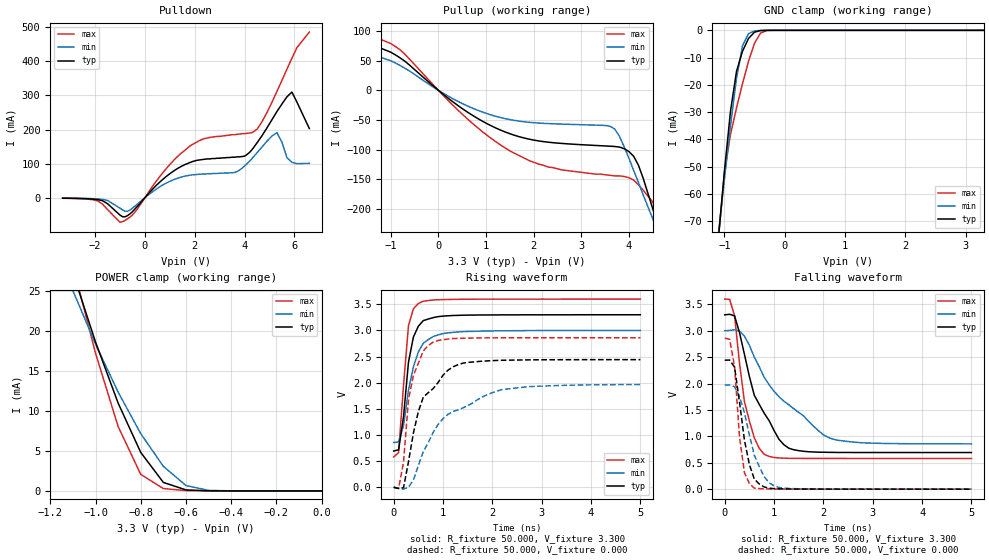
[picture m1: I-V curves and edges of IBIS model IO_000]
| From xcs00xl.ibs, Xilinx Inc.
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|   Model IO_000
[Model]   IO_000
Model_type   I/O
Polarity   Non-Inverting
Enable   Active-Low
Vinl =   0.800V
Vinh =   2.000V
Vmeas =   1.650V
Cref =  50.000pF
Rref =   1.000M
Vref =  0.000V
C_comp   5.300pF   3.500pF   6.800pF
[Temperature Range]   50.000   100.000   0.000
[Voltage Range]   3.300V   3.000V   3.600V
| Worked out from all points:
|   slope of the pulldown table from 0 to 0.495 V, typ, clamps not added: 12.8 ohm
|   slope of the pullup table from 0 to 0.495 V, typ, clamps not added: 16.3 ohm
|   GND clamp passes 1 mA (typ) near -0.52 V on its own axis
|   POWER clamp passes 1 mA (typ) near -0.69 V on its own axis
|   rising waveform, R_fixture 50.000, V_fixture 3.300: 20-80 % time 202ps typ, 279ps min, 151ps max; typ from 0.693 V to 3.3 V
|   rising waveform, R_fixture 50.000, V_fixture 0.000: 20-80 % time 556ps typ, 1.03ns min, 256ps max; typ from 0 V to 2.44 V
|   falling waveform, R_fixture 50.000, V_fixture 3.300: 20-80 % time 599ps typ, 1.13ns min, 301ps max; typ from 3.3 V to 0.694 V
|   falling waveform, R_fixture 50.000, V_fixture 0.000: 20-80 % time 241ps typ, 361ps min, 159ps max; typ from 2.44 V to 0.001 V
[Pulldown]
| voltage   I(typ)   I(min)   I(max)
-3.3V     -1.3mA     -1mA       -1.5mA
-1.9V     -5.4mA     -3.4mA     -9mA
-1V       -50.64mA   -30.43mA   -71.65mA
-700mV    -52.55mA   -39.74mA   -61.89mA
800mV     58.88mA    40.69mA    80.44mA
1.8V      103mA      66.09mA    151mA
3.6V      119mA      74.19mA    185mA
4V        122mA      93.03mA    188mA
4.5V      161mA      132mA      201mA
5.3V      253mA      191mA      312mA
5.9V      310mA      104mA      409mA
6.6V      203mA      101mA      486mA
[Pullup]
| voltage   I(typ)   I(min)   I(max)
-3.3V     5.1mA      940uA      37.2mA
-3.1V     7.54mA     1.17mA     90.7mA
-2.9V     27.6mA     1.66mA     104mA
-2.7V     86.4mA     3.45mA     105mA
-2.3V     90.2mA     70mA       105mA
-1.5V     80.17mA    63.43mA    95.35mA
-800mV    54.4mA     41.67mA    67.93mA
1.5V      -72.97mA   -49.19mA   -102mA
3.7V      -94.47mA   -64.95mA   -144mA
4.1V      -111mA     -135mA     -151mA
4.7V      -250mA     -255mA     -227mA
6.6V      -645mA     -572mA     -737mA
[GND_clamp]
| voltage   I(typ)   I(min)   I(max)
-3.3V     -539mA     -461mA     -635mA
-1.1V     -76.29mA   -74.81mA   -76.3mA
-1V       -51.66mA   -54.6mA    -52.25mA
-900mV    -29.77mA   -35.09mA   -38.23mA
-800mV    -15.1mA    -17.65mA   -28.49mA
-700mV    -7.645mA   -5.66mA    -19.53mA
-600mV    -2.968mA   -1.205mA   -11.34mA
-500mV    -649uA     -202uA     -4.68mA
-400mV    -83.34uA   -28.89uA   -976uA
-300mV    -8.303uA   -3.567uA   -95.2uA
3.3V      90.24nA    487nA      4.544uA
[POWER_clamp]
| voltage   I(typ)   I(min)   I(max)
-3.3V     51.86mA    10.89mA    181mA
-3.1V     70.08mA    13.61mA    230mA
-3V       85.17mA    15.89mA    249mA
-2.9V     108mA      19.33mA    255mA
-2.8V     138mA      24.96mA    249mA
-1.1V     27.32mA    25.08mA    28.22mA
-1V       18.65mA    18.39mA    17.25mA
-900mV    11mA       12.37mA    8.069mA
-800mV    4.821mA    7.171mA    2.071mA
-700mV    1.064mA    3.083mA    296uA
-600mV    127uA      671uA      39.67uA
0V        90.2nA     23.32nA    5.636uA
[Ramp]
| variable   typ   min   max
dV/dt_r   1.464/0.539n   1.179/1.025n   1.715/0.284n
dV/dt_f   1.563/0.572n   1.285/1.103n   1.810/0.310n
R_load = 50.000
[Rising Waveform]
R_fixture = 50.000
V_fixture = 3.300
V_fixture_min = 3.000
V_fixture_max = 3.600
L_fixture = 0.000H
C_fixture = 0.000F
| time   V(typ)   V(min)   V(max)
0s        693mV      856mV      580mV
100ps     716mV      866mV      662mV
200ps     1.348V     1.178V     1.949V
300ps     2.389V     1.855V     3.087V
400ps     2.871V     2.303V     3.412V
500ps     3.078V     2.585V     3.514V
600ps     3.186V     2.752V     3.557V
800ps     3.243V     2.881V     3.58V
1.2ns     3.284V     2.961V     3.592V
5ns       3.298V     2.998V     3.598V
[Rising Waveform]
R_fixture = 50.000
V_fixture = 0.000
V_fixture_min = 0.000
V_fixture_max = 0.000
L_fixture = 0.000H
C_fixture = 0.000F
| time   V(typ)   V(min)   V(max)
0s        0V         0V         0V
100ps     -23.77mV   -15.72mV   -21.66mV
200ps     -8.12mV    -35.98mV   481mV
300ps     485mV      1.41mV     1.671V
400ps     1.037V     139mV      2.141V
600ps     1.722V     682mV      2.607V
800ps     1.886V     1.047V     2.775V
1.3ns     2.341V     1.479V     2.846V
2.2ns     2.428V     1.869V     2.858V
5ns       2.44V      1.965V     2.859V
[Falling Waveform]
R_fixture = 50.000
V_fixture = 3.300
V_fixture_min = 3.000
V_fixture_max = 3.600
L_fixture = 0.000H
C_fixture = 0.000F
| time   V(typ)   V(min)   V(max)
0s        3.3V       3V         3.599V
100ps     3.311V     3.005V     3.594V
200ps     3.281V     3.018V     3.286V
400ps     2.552V     2.897V     1.658V
600ps     1.778V     2.501V     972mV
800ps     1.439V     2.118V     661mV
1.1ns     946mV      1.751V     592mV
1.3ns     776mV      1.599V     585mV
2.2ns     697mV      946mV      583mV
5ns       694mV      858mV      582mV
[Falling Waveform]
R_fixture = 50.000
V_fixture = 0.000
V_fixture_min = 0.000
V_fixture_max = 0.000
L_fixture = 0.000H
C_fixture = 0.000F
| time   V(typ)   V(min)   V(max)
0s        2.442V     1.97V      2.861V
100ps     2.445V     1.971V     2.837V
200ps     2.311V     1.94V      2.325V
300ps     1.651V     1.75V      989mV
400ps     930mV      1.45V      315mV
500ps     468mV      1.027V     107mV
600ps     193mV      643mV      20.71mV
800ps     42.81mV    237mV      6.543mV
1.1ns     7.379mV    34.23mV    3.456mV
5ns       1.154mV    1.175mV    1.068mV
